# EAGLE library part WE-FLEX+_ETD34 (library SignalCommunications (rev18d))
WE-FLEX+ Flexible Transformer for DC/DC Converter Characteristics Transformer with 6 identical windings Power up to 300 W possible Isolation voltage 500 VDC Low leakage inductance Operating temperature: –40 °C to +125 °C Applications All kind of switching regulators -Flyback converters -Forward converters -Push-pull converters -Step-up/step-down converters -SEPIC converter Details see: http://katalog.we-online.de/en/pbs/WE-FLEX-PLUS Updated by Dan Xu 2014-07-07 2014 (C) Wurth Elektronik
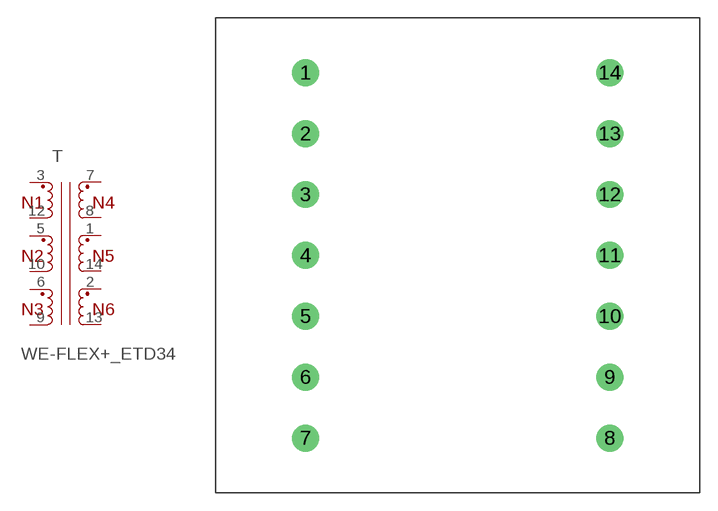
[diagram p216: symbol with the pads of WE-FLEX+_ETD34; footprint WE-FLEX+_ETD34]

Designator prefix T

## WE-FLEX+_ETD34_749197201, WE-FLEX+_ETD34_749197211, WE-FLEX+_ETD34_749197221, WE-FLEX+_ETD34_749197231, WE-FLEX+_ETD34_749197241  [WE-FLEX+_ETD34]
1  4  pas
2  6  pas
3  1  pas
5  11  pas
6  9  pas
7  2  pas
8  3  pas
9  8  pas
10  10  pas
12  12  pas
13  7  pas
14  5  pas

## Footprint WE-FLEX+_ETD34 (pad centres in mm)
Transformer, ETD34 THT 14Pin
drill 1.5: 1 -12.7,15.24; 2 -12.7,10.16; 3 -12.7,5.08; 4 -12.7,0; 5 -12.7,-5.08; 6 -12.7,-10.16; 7 -12.7,-15.24; 8 12.7,-15.24; 9 12.7,-10.16; 10 12.7,-5.08; 11 12.7,0; 12 12.7,5.08; 13 12.7,10.16; 14 12.7,15.24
